(* Logix 5000 AddOnInstructionDefinition export Banner_QS18E_Param_v3; software revision 30.00; part 2 of 3 *)
(* tags used below, declared in another part *)
   QS18E : Banner_QS18E_v3;
   Port_Data : Banner_IOL_Port_v2;
   Port : DINT;
   Sensor_Type : DINT;   // 1 = D, DV, LP, CV, & FP models, 2 = EV or E models, 3 = RV or R models.
   Local_Control : DINT;
   Command_Being_Processed : BOOL;
   Update_Archive : BOOL;
   Index_Write_Inprocess : INT;
   Index_Write_Control : INT;
   Inprocess_Index : DINT;
(* Banner_QS18E_Param_v3, continued *)

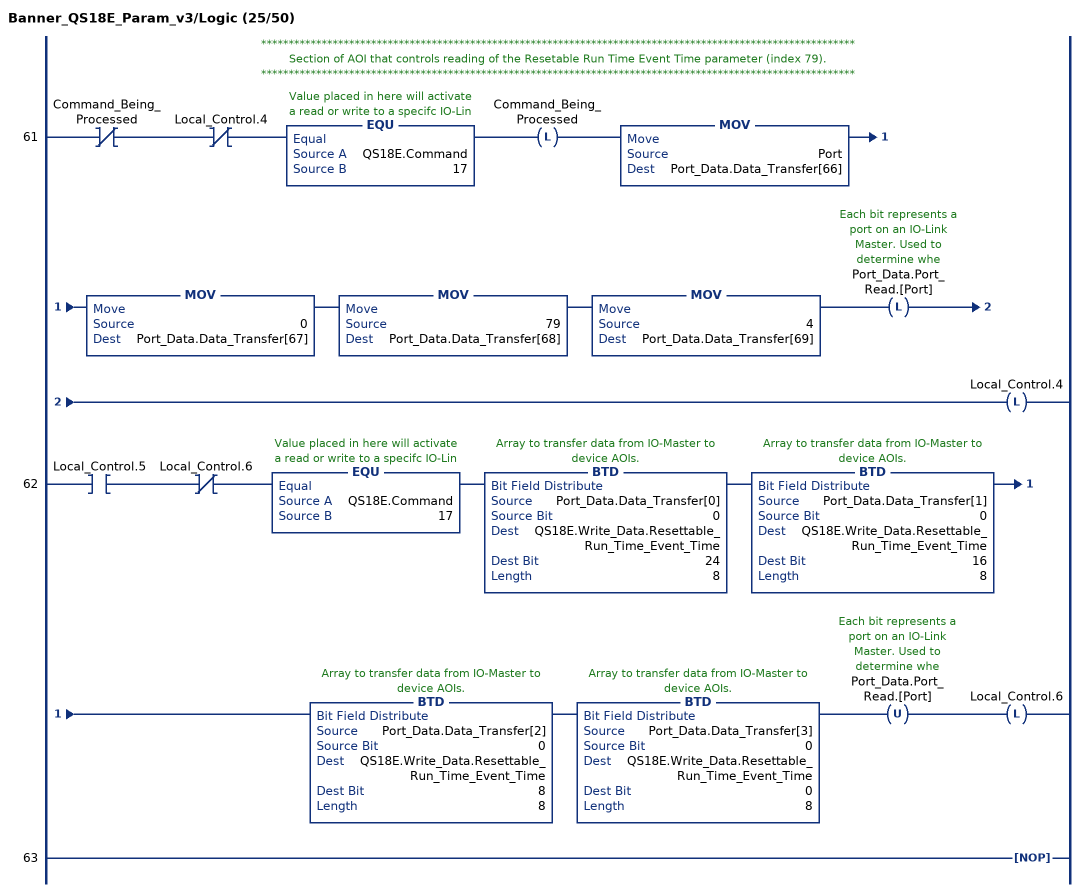
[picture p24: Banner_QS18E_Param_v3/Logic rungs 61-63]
   // ************************************************************************************************************
   // Section of AOI that controls reading of the Resetable Run Time Event Time parameter (index 79).
   // ************************************************************************************************************
   61: XIO(Command_Being_Processed)XIO(Local_Control.4)EQU(QS18E.Command,17)OTL(Command_Being_Processed)MOV(Port,Port_Data.Data_Transfer[66])MOV(0,Port_Data.Data_Transfer[67])MOV(79,Port_Data.Data_Transfer[68])MOV(4,Port_Data.Data_Transfer[69])OTL(Port_Data.Port_Read.[Port])OTL(Local_Control.4);
   62: XIC(Local_Control.5)XIO(Local_Control.6)EQU(QS18E.Command,17)BTD(Port_Data.Data_Transfer[0],0,QS18E.Write_Data.Resettable_Run_Time_Event_Time,24,8)BTD(Port_Data.Data_Transfer[1],0,QS18E.Write_Data.Resettable_Run_Time_Event_Time,16,8)BTD(Port_Data.Data_Transfer[2],0,QS18E.Write_Data.Resettable_Run_Time_Event_Time,8,8)BTD(Port_Data.Data_Transfer[3],0,QS18E.Write_Data.Resettable_Run_Time_Event_Time,0,8)OTU(Port_Data.Port_Read.[Port])OTL(Local_Control.6);
   63: NOP();
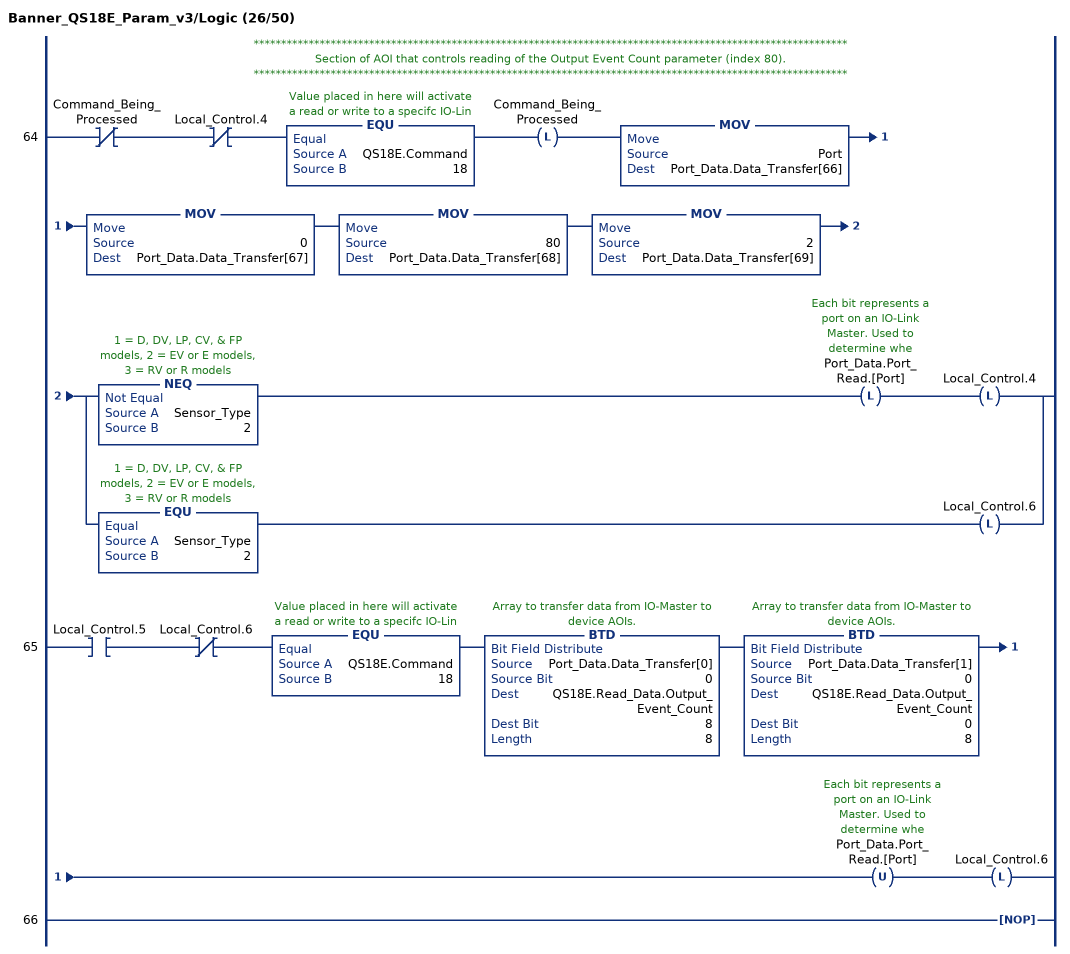
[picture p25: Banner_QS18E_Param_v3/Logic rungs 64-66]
   // ************************************************************************************************************
   // Section of AOI that controls reading of the Output Event Count parameter (index 80).
   // ************************************************************************************************************
   64: XIO(Command_Being_Processed)XIO(Local_Control.4)EQU(QS18E.Command,18)OTL(Command_Being_Processed)MOV(Port,Port_Data.Data_Transfer[66])MOV(0,Port_Data.Data_Transfer[67])MOV(80,Port_Data.Data_Transfer[68])MOV(2,Port_Data.Data_Transfer[69])[NEQ(Sensor_Type,2) OTL(Port_Data.Port_Read.[Port]) OTL(Local_Control.4) ,EQU(Sensor_Type,2) OTL(Local_Control.6) ];
   65: XIC(Local_Control.5)XIO(Local_Control.6)EQU(QS18E.Command,18)BTD(Port_Data.Data_Transfer[0],0,QS18E.Read_Data.Output_Event_Count,8,8)BTD(Port_Data.Data_Transfer[1],0,QS18E.Read_Data.Output_Event_Count,0,8)OTU(Port_Data.Port_Read.[Port])OTL(Local_Control.6);
   66: NOP();
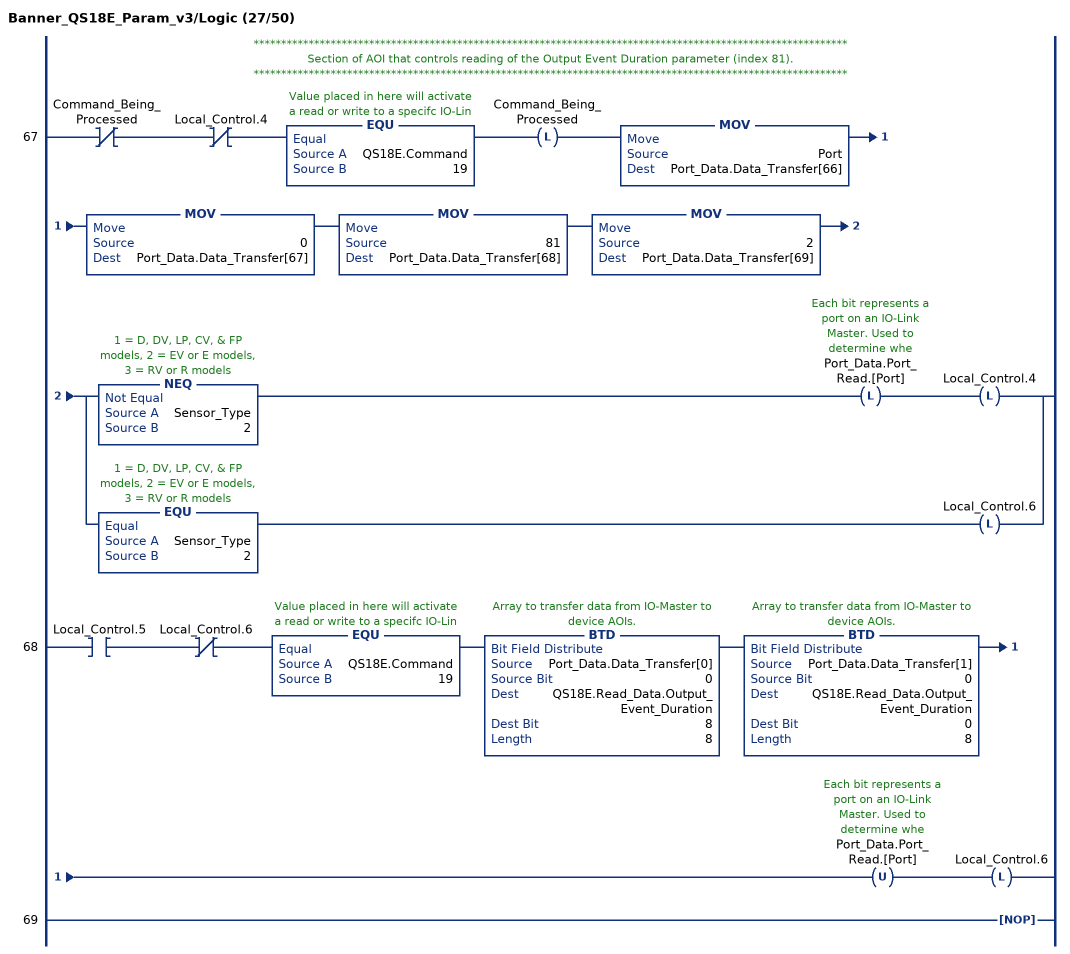
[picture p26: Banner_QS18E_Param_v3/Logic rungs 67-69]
   // ************************************************************************************************************
   // Section of AOI that controls reading of the Output Event Duration parameter (index 81).
   // ************************************************************************************************************
   67: XIO(Command_Being_Processed)XIO(Local_Control.4)EQU(QS18E.Command,19)OTL(Command_Being_Processed)MOV(Port,Port_Data.Data_Transfer[66])MOV(0,Port_Data.Data_Transfer[67])MOV(81,Port_Data.Data_Transfer[68])MOV(2,Port_Data.Data_Transfer[69])[NEQ(Sensor_Type,2) OTL(Port_Data.Port_Read.[Port]) OTL(Local_Control.4) ,EQU(Sensor_Type,2) OTL(Local_Control.6) ];
   68: XIC(Local_Control.5)XIO(Local_Control.6)EQU(QS18E.Command,19)BTD(Port_Data.Data_Transfer[0],0,QS18E.Read_Data.Output_Event_Duration,8,8)BTD(Port_Data.Data_Transfer[1],0,QS18E.Read_Data.Output_Event_Duration,0,8)OTU(Port_Data.Port_Read.[Port])OTL(Local_Control.6);
   69: NOP();
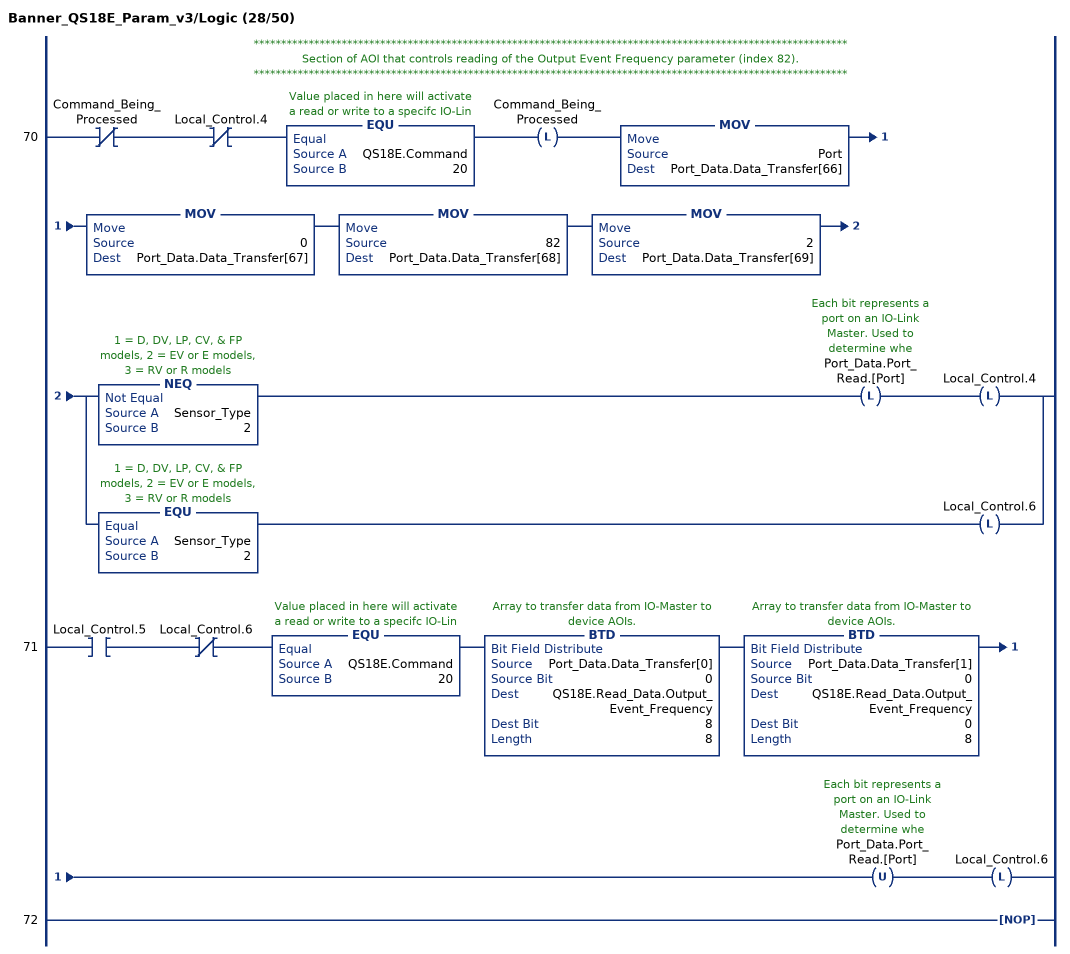
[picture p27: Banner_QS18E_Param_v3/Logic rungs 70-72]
   // ************************************************************************************************************
   // Section of AOI that controls reading of the Output Event Frequency parameter (index 82).
   // ************************************************************************************************************
   70: XIO(Command_Being_Processed)XIO(Local_Control.4)EQU(QS18E.Command,20)OTL(Command_Being_Processed)MOV(Port,Port_Data.Data_Transfer[66])MOV(0,Port_Data.Data_Transfer[67])MOV(82,Port_Data.Data_Transfer[68])MOV(2,Port_Data.Data_Transfer[69])[NEQ(Sensor_Type,2) OTL(Port_Data.Port_Read.[Port]) OTL(Local_Control.4) ,EQU(Sensor_Type,2) OTL(Local_Control.6) ];
   71: XIC(Local_Control.5)XIO(Local_Control.6)EQU(QS18E.Command,20)BTD(Port_Data.Data_Transfer[0],0,QS18E.Read_Data.Output_Event_Frequency,8,8)BTD(Port_Data.Data_Transfer[1],0,QS18E.Read_Data.Output_Event_Frequency,0,8)OTU(Port_Data.Port_Read.[Port])OTL(Local_Control.6);
   72: NOP();
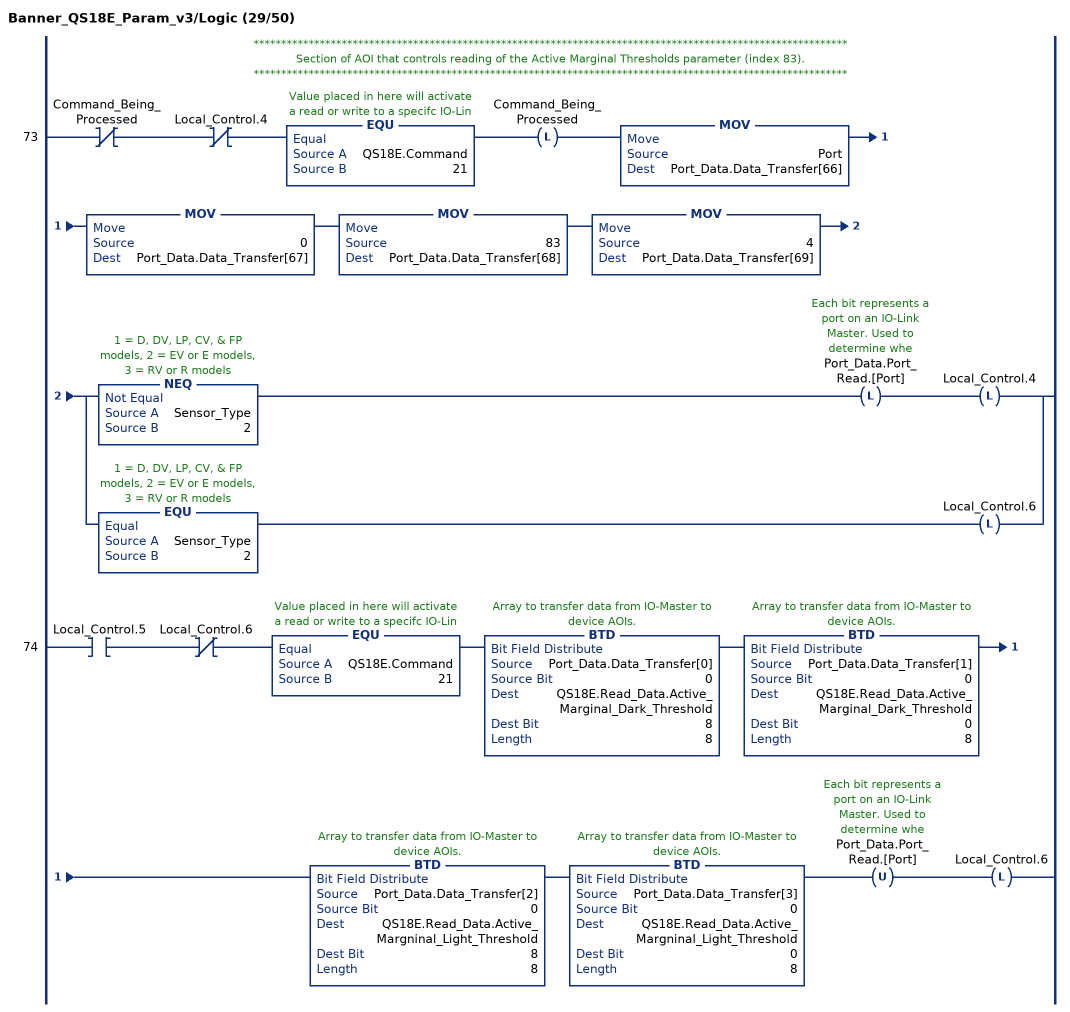
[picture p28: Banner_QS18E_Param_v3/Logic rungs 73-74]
   // ************************************************************************************************************
   // Section of AOI that controls reading of the Active Marginal Thresholds parameter (index 83).
   // ************************************************************************************************************
   73: XIO(Command_Being_Processed)XIO(Local_Control.4)EQU(QS18E.Command,21)OTL(Command_Being_Processed)MOV(Port,Port_Data.Data_Transfer[66])MOV(0,Port_Data.Data_Transfer[67])MOV(83,Port_Data.Data_Transfer[68])MOV(4,Port_Data.Data_Transfer[69])[NEQ(Sensor_Type,2) OTL(Port_Data.Port_Read.[Port]) OTL(Local_Control.4) ,EQU(Sensor_Type,2) OTL(Local_Control.6) ];
   74: XIC(Local_Control.5)XIO(Local_Control.6)EQU(QS18E.Command,21)BTD(Port_Data.Data_Transfer[0],0,QS18E.Read_Data.Active_Marginal_Dark_Threshold,8,8)BTD(Port_Data.Data_Transfer[1],0,QS18E.Read_Data.Active_Marginal_Dark_Threshold,0,8)BTD(Port_Data.Data_Transfer[2],0,QS18E.Read_Data.Active_Margninal_Light_Threshold,8,8)BTD(Port_Data.Data_Transfer[3],0,QS18E.Read_Data.Active_Margninal_Light_Threshold,0,8)OTU(Port_Data.Port_Read.[Port])OTL(Local_Control.6);
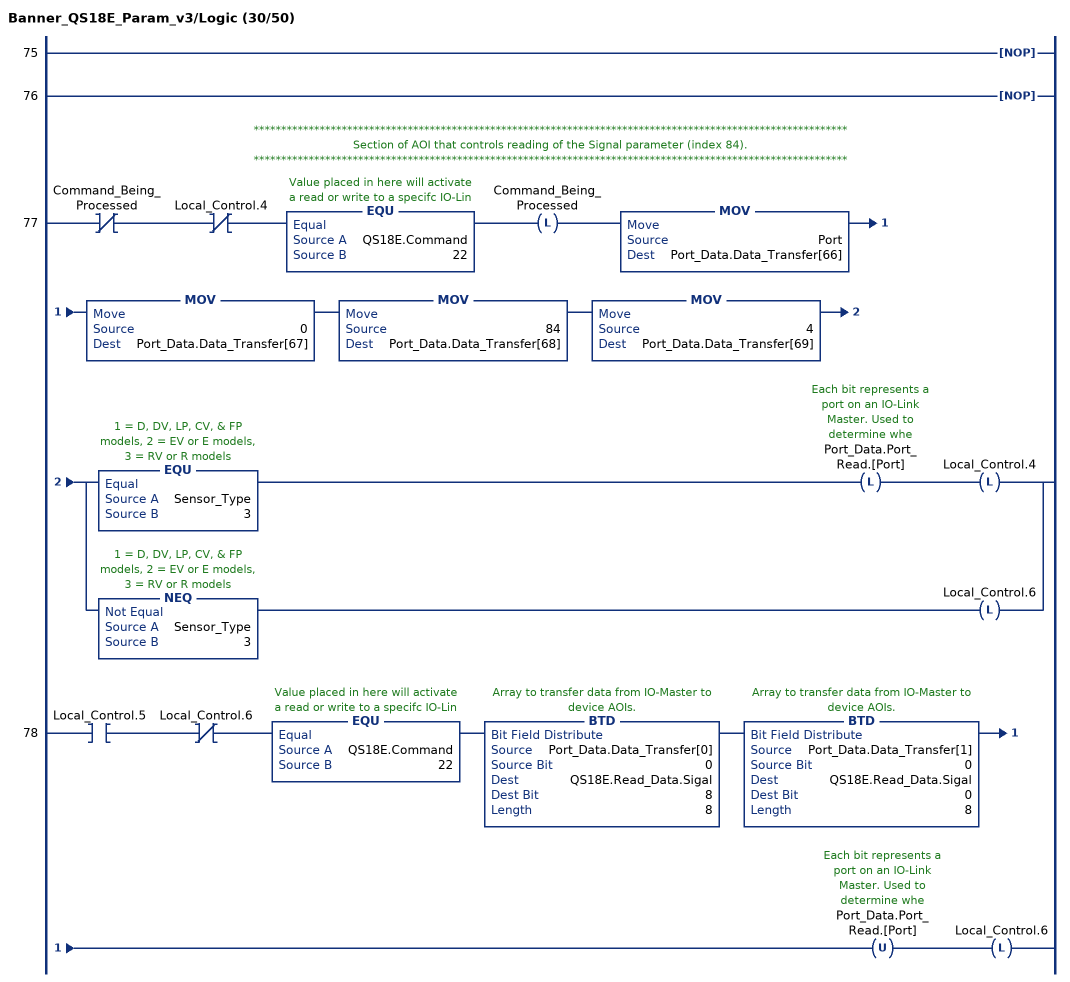
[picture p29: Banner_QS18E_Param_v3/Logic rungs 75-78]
   75: NOP();
   76: NOP();
   // ************************************************************************************************************
   // Section of AOI that controls reading of the Signal parameter (index 84).
   // ************************************************************************************************************
   77: XIO(Command_Being_Processed)XIO(Local_Control.4)EQU(QS18E.Command,22)OTL(Command_Being_Processed)MOV(Port,Port_Data.Data_Transfer[66])MOV(0,Port_Data.Data_Transfer[67])MOV(84,Port_Data.Data_Transfer[68])MOV(4,Port_Data.Data_Transfer[69])[EQU(Sensor_Type,3) OTL(Port_Data.Port_Read.[Port]) OTL(Local_Control.4) ,NEQ(Sensor_Type,3) OTL(Local_Control.6) ];
   78: XIC(Local_Control.5)XIO(Local_Control.6)EQU(QS18E.Command,22)BTD(Port_Data.Data_Transfer[0],0,QS18E.Read_Data.Sigal,8,8)BTD(Port_Data.Data_Transfer[1],0,QS18E.Read_Data.Sigal,0,8)OTU(Port_Data.Port_Read.[Port])OTL(Local_Control.6);
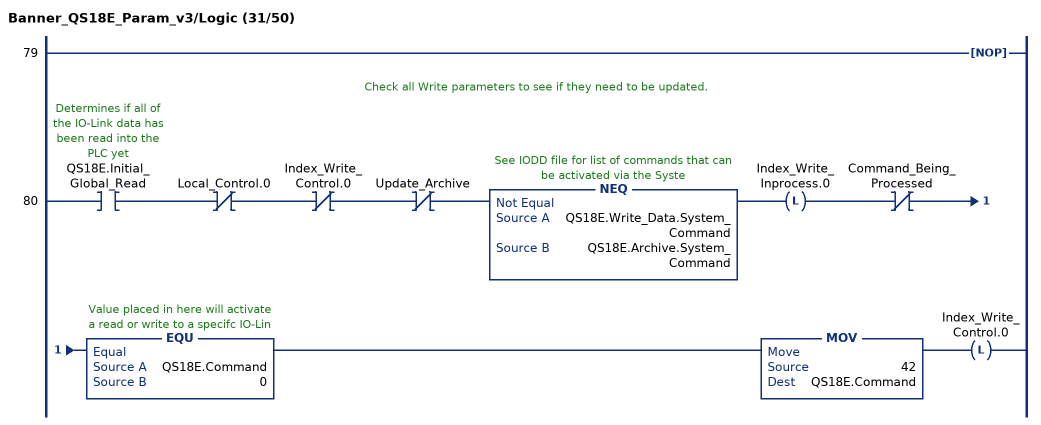
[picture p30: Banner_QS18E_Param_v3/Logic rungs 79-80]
   79: NOP();
   // Check all Write parameters to see if they need to be updated.
   80: XIC(QS18E.Initial_Global_Read)XIO(Local_Control.0)XIO(Index_Write_Control.0)XIO(Update_Archive)NEQ(QS18E.Write_Data.System_Command,QS18E.Archive.System_Command)OTL(Index_Write_Inprocess.0)XIO(Command_Being_Processed)EQU(QS18E.Command,0)MOV(42,QS18E.Command)OTL(Index_Write_Control.0);
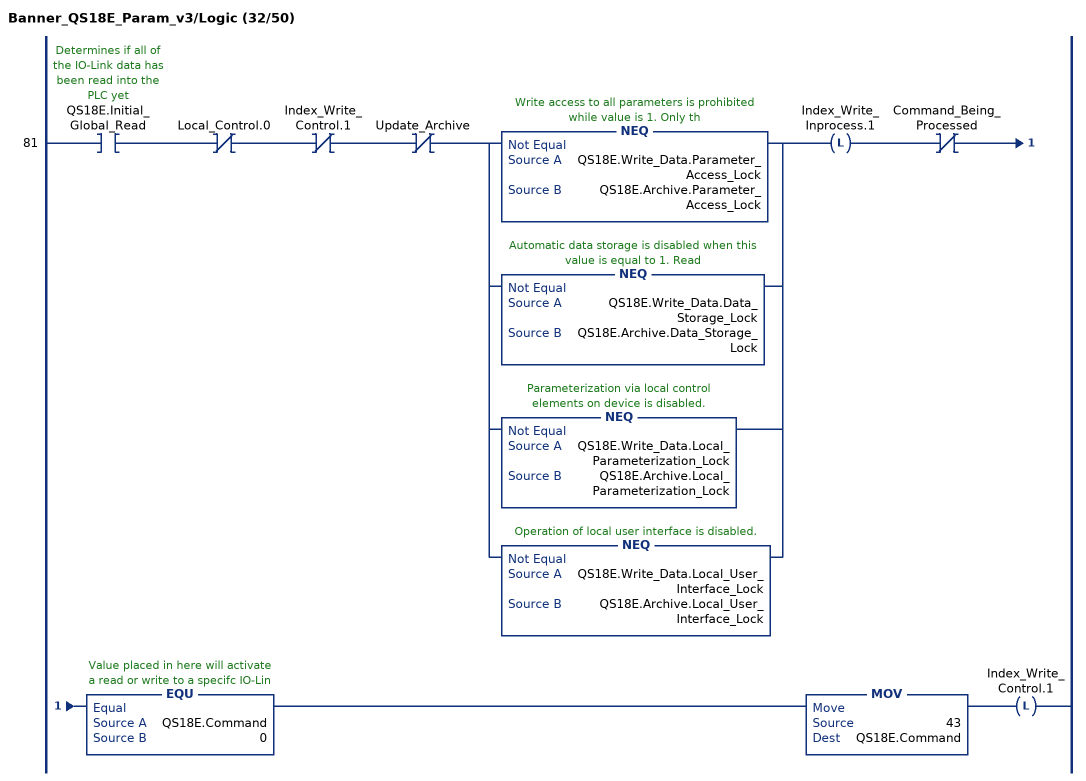
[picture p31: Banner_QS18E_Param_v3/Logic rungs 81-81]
   81: XIC(QS18E.Initial_Global_Read)XIO(Local_Control.0)XIO(Index_Write_Control.1)XIO(Update_Archive)[NEQ(QS18E.Write_Data.Parameter_Access_Lock,QS18E.Archive.Parameter_Access_Lock) ,NEQ(QS18E.Write_Data.Data_Storage_Lock,QS18E.Archive.Data_Storage_Lock) ,NEQ(QS18E.Write_Data.Local_Parameterization_Lock,QS18E.Archive.Local_Parameterization_Lock) ,NEQ(QS18E.Write_Data.Local_User_Interface_Lock,QS18E.Archive.Local_User_Interface_Lock) ]OTL(Index_Write_Inprocess.1)XIO(Command_Being_Processed)EQU(QS18E.Command,0)MOV(43,QS18E.Command)OTL(Index_Write_Control.1);
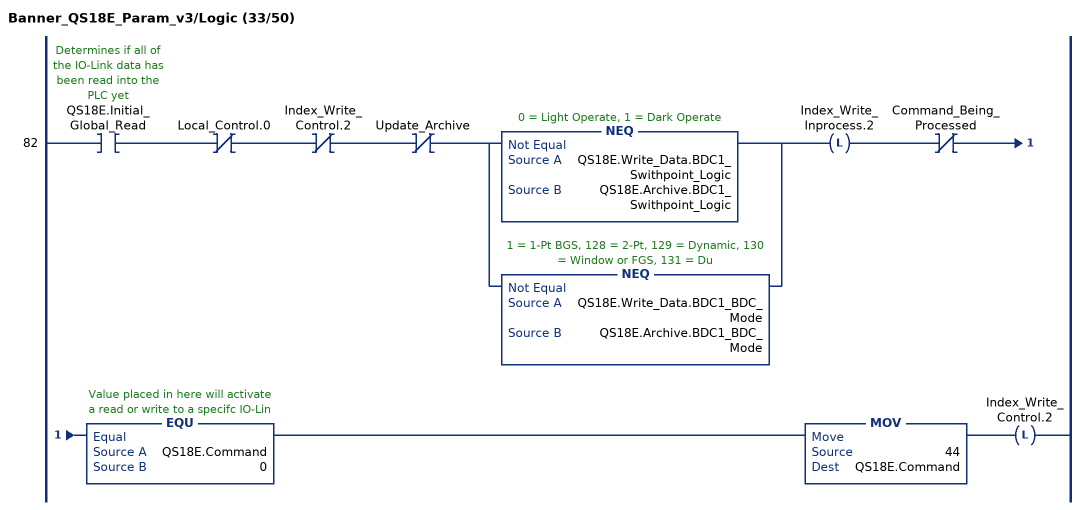
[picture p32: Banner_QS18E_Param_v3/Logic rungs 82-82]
   82: XIC(QS18E.Initial_Global_Read)XIO(Local_Control.0)XIO(Index_Write_Control.2)XIO(Update_Archive)[NEQ(QS18E.Write_Data.BDC1_Swithpoint_Logic,QS18E.Archive.BDC1_Swithpoint_Logic) ,NEQ(QS18E.Write_Data.BDC1_BDC_Mode,QS18E.Archive.BDC1_BDC_Mode) ]OTL(Index_Write_Inprocess.2)XIO(Command_Being_Processed)EQU(QS18E.Command,0)MOV(44,QS18E.Command)OTL(Index_Write_Control.2);
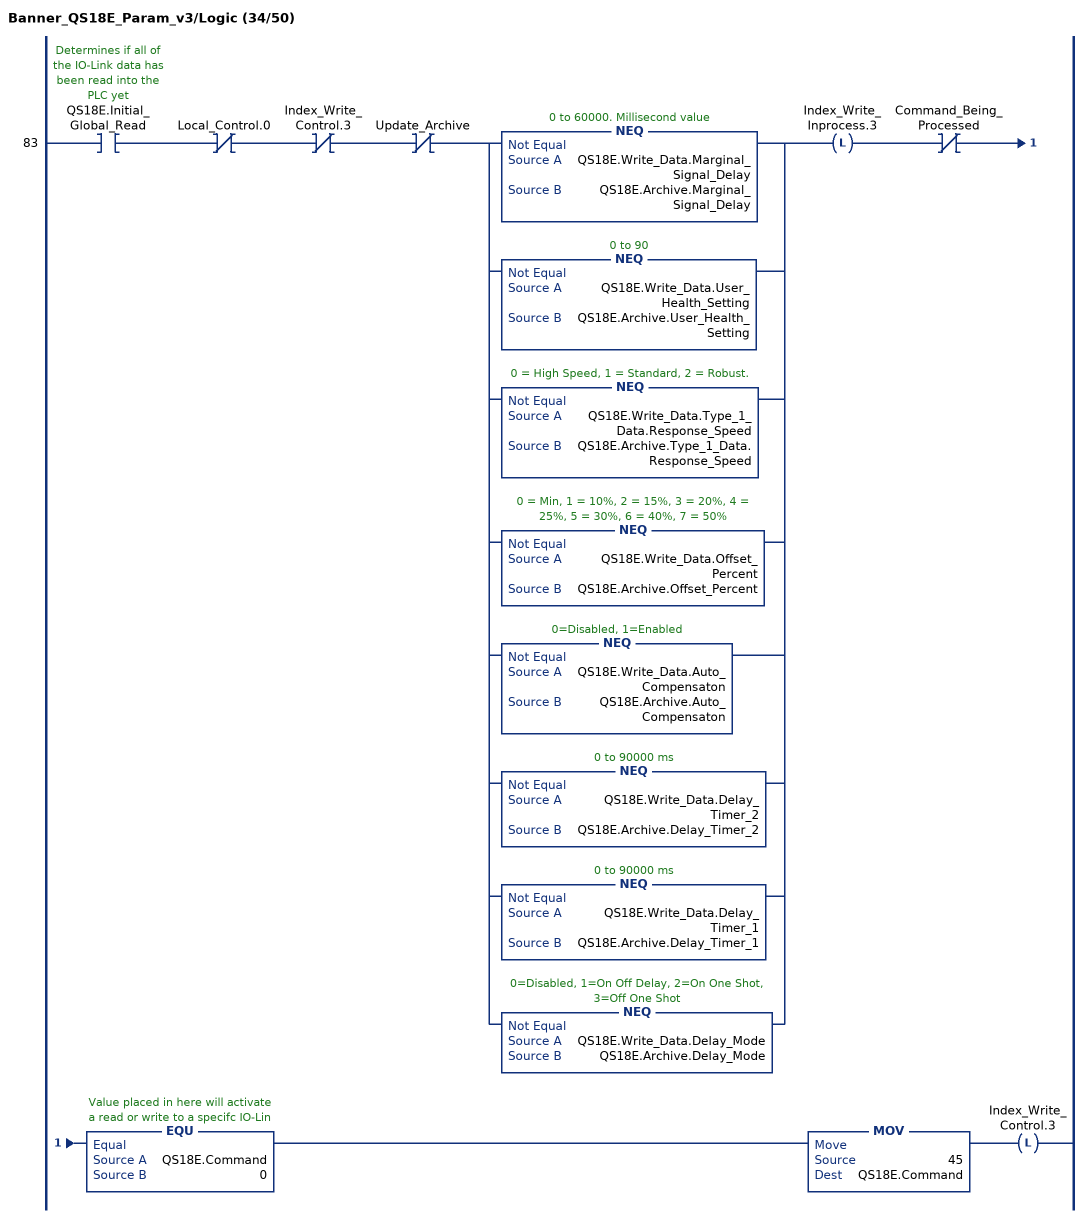
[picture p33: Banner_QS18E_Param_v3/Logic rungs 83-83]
   83: XIC(QS18E.Initial_Global_Read)XIO(Local_Control.0)XIO(Index_Write_Control.3)XIO(Update_Archive)[NEQ(QS18E.Write_Data.Marginal_Signal_Delay,QS18E.Archive.Marginal_Signal_Delay) ,NEQ(QS18E.Write_Data.User_Health_Setting,QS18E.Archive.User_Health_Setting) ,NEQ(QS18E.Write_Data.Type_1_Data.Response_Speed,QS18E.Archive.Type_1_Data.Response_Speed) ,NEQ(QS18E.Write_Data.Offset_Percent,QS18E.Archive.Offset_Percent) ,NEQ(QS18E.Write_Data.Auto_Compensaton,QS18E.Archive.Auto_Compensaton) ,NEQ(QS18E.Write_Data.Delay_Timer_2,QS18E.Archive.Delay_Timer_2) ,NEQ(QS18E.Write_Data.Delay_Timer_1,QS18E.Archive.Delay_Timer_1) ,NEQ(QS18E.Write_Data.Delay_Mode,QS18E.Archive.Delay_Mode) ]OTL(Index_Write_Inprocess.3)XIO(Command_Being_Processed)EQU(QS18E.Command,0)MOV(45,QS18E.Command)OTL(Index_Write_Control.3);
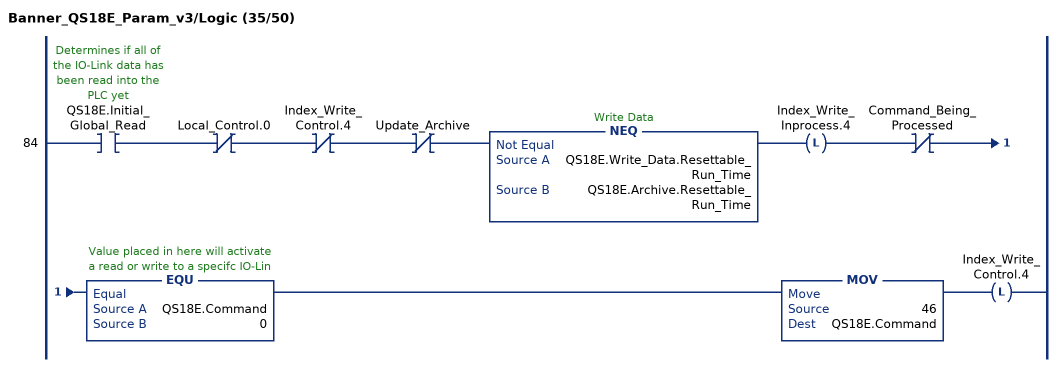
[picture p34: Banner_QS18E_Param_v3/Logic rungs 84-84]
   84: XIC(QS18E.Initial_Global_Read)XIO(Local_Control.0)XIO(Index_Write_Control.4)XIO(Update_Archive)NEQ(QS18E.Write_Data.Resettable_Run_Time,QS18E.Archive.Resettable_Run_Time)OTL(Index_Write_Inprocess.4)XIO(Command_Being_Processed)EQU(QS18E.Command,0)MOV(46,QS18E.Command)OTL(Index_Write_Control.4);
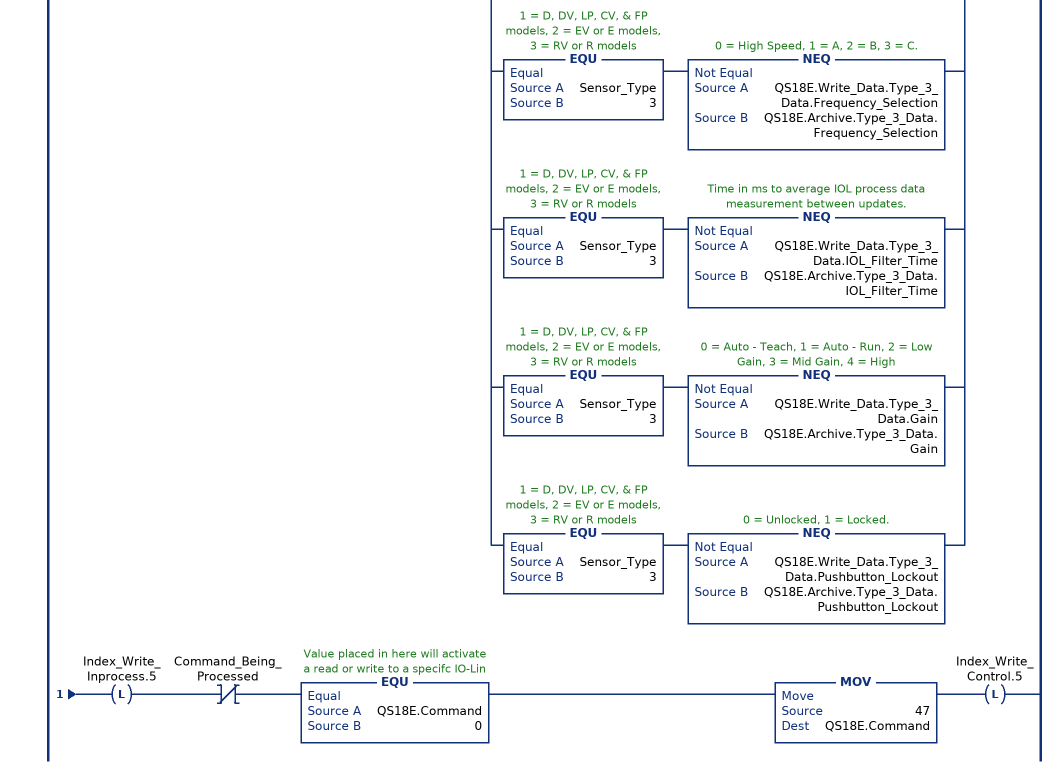
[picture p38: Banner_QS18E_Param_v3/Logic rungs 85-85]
   85: XIC(QS18E.Initial_Global_Read)XIO(Local_Control.0)XIO(Index_Write_Control.5)XIO(Update_Archive)[EQU(Sensor_Type,1) NEQ(QS18E.Write_Data.Type_1_Data.Polarity_of_Pins_2_and_4,QS18E.Archive.Type_1_Data.Polarity_of_Pins_2_and_4) ,EQU(Sensor_Type,1) NEQ(QS18E.Write_Data.Type_1_Data.Pin_2_Config,QS18E.Archive.Type_1_Data.Pin_2_Config) ,EQU(Sensor_Type,1) NEQ(QS18E.Write_Data.Type_1_Data.Process_Data_Input_Config,QS18E.Archive.Type_1_Data.Process_Data_Input_Config) ,EQU(Sensor_Type,1) NEQ(QS18E.Write_Data.Type_1_Data.Marginal_Mode,QS18E.Archive.Type_1_Data.Marginal_Mode) ,EQU(Sensor_Type,1) NEQ(QS18E.Write_Data.Type_1_Data.User_Marginal_Light,QS18E.Archive.Type_1_Data.User_Marginal_Light) ,EQU(Sensor_Type,1) NEQ(QS18E.Write_Data.Type_1_Data.User_Marginal_Dark,QS18E.Archive.Type_1_Data.User_Marginal_Dark) ,EQU(Sensor_Type,1) NEQ(QS18E.Write_Data.Type_1_Data.LED_Power,QS18E.Archive.Type_1_Data.LED_Power) ,EQU(Sensor_Type,2) NEQ(QS18E.Write_Data.Type_2_Data.Polarity_of_Pins_2_and_4,QS18E.Archive.Type_2_Data.Polarity_of_Pins_2_and_4) ,EQU(Sensor_Type,2) NEQ(QS18E.Write_Data.Type_2_Data.Pin_2_Config,QS18E.Archive.Type_2_Data.Pin_2_Config) ,EQU(Sensor_Type,2) NEQ(QS18E.Write_Data.Type_2_Data.Frequency_Selection,QS18E.Archive.Type_2_Data.Frequency_Selection) ,EQU(Sensor_Type,2) NEQ(QS18E.Write_Data.Type_2_Data.Power_Level,QS18E.Archive.Type_2_Data.Power_Level) ,EQU(Sensor_Type,2) NEQ(QS18E.Write_Data.Type_2_Data.Pushbutton_Lockout,QS18E.Archive.Type_2_Data.Pushbutton_Lockout) ,EQU(Sensor_Type,3) NEQ(QS18E.Write_Data.Type_3_Data.Polarity_of_Pins_2_and_4,QS18E.Archive.Type_3_Data.Polarity_of_Pins_2_and_4) ,EQU(Sensor_Type,3) NEQ(QS18E.Write_Data.Type_3_Data.Pin_2_Config,QS18E.Archive.Type_3_Data.Pin_2_Config) ,EQU(Sensor_Type,3) NEQ(QS18E.Write_Data.Type_3_Data.Process_Data_Input_Config,QS18E.Archive.Type_3_Data.Process_Data_Input_Config) ,EQU(Sensor_Type,3) NEQ(QS18E.Write_Data.Type_3_Data.Marginal_Mode,QS18E.Archive.Type_3_Data.Marginal_Mode) ,EQU(Sensor_Type,3) NEQ(QS18E.Write_Data.Type_3_Data.User_Marginal_Light,QS18E.Archive.Type_3_Data.User_Marginal_Light) ,EQU(Sensor_Type,3) NEQ(QS18E.Write_Data.Type_3_Data.User_Marginal_Dark,QS18E.Archive.Type_3_Data.User_Marginal_Dark) ,EQU(Sensor_Type,3) NEQ(QS18E.Write_Data.Type_3_Data.Frequency_Selection,QS18E.Archive.Type_3_Data.Frequency_Selection) ,EQU(Sensor_Type,3) NEQ(QS18E.Write_Data.Type_3_Data.IOL_Filter_Time,QS18E.Archive.Type_3_Data.IOL_Filter_Time) ,EQU(Sensor_Type,3) NEQ(QS18E.Write_Data.Type_3_Data.Gain,QS18E.Archive.Type_3_Data.Gain) ,EQU(Sensor_Type,3) NEQ(QS18E.Write_Data.Type_3_Data.Pushbutton_Lockout,QS18E.Archive.Type_3_Data.Pushbutton_Lockout) ]OTL(Index_Write_Inprocess.5)XIO(Command_Being_Processed)EQU(QS18E.Command,0)MOV(47,QS18E.Command)OTL(Index_Write_Control.5);
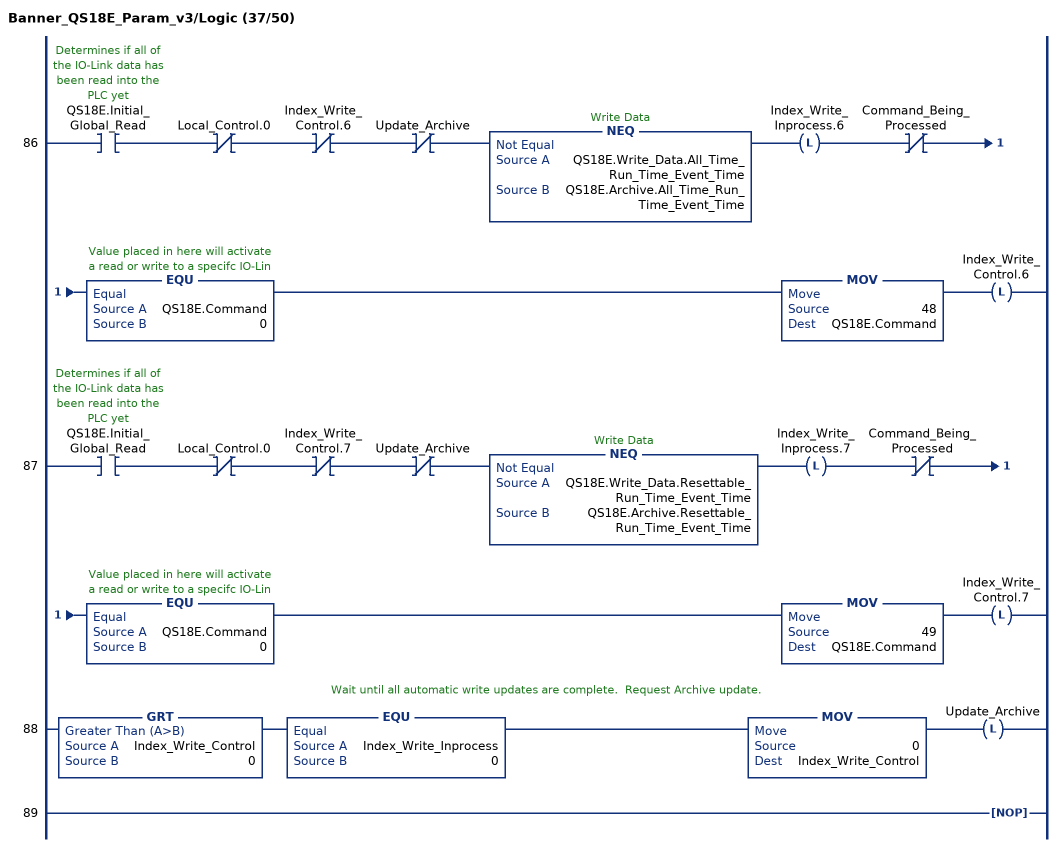
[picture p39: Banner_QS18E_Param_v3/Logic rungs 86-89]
   86: XIC(QS18E.Initial_Global_Read)XIO(Local_Control.0)XIO(Index_Write_Control.6)XIO(Update_Archive)NEQ(QS18E.Write_Data.All_Time_Run_Time_Event_Time,QS18E.Archive.All_Time_Run_Time_Event_Time)OTL(Index_Write_Inprocess.6)XIO(Command_Being_Processed)EQU(QS18E.Command,0)MOV(48,QS18E.Command)OTL(Index_Write_Control.6);
   87: XIC(QS18E.Initial_Global_Read)XIO(Local_Control.0)XIO(Index_Write_Control.7)XIO(Update_Archive)NEQ(QS18E.Write_Data.Resettable_Run_Time_Event_Time,QS18E.Archive.Resettable_Run_Time_Event_Time)OTL(Index_Write_Inprocess.7)XIO(Command_Being_Processed)EQU(QS18E.Command,0)MOV(49,QS18E.Command)OTL(Index_Write_Control.7);
   // Wait until all automatic write updates are complete.  Request Archive update.
   88: GRT(Index_Write_Control,0)EQU(Index_Write_Inprocess,0)MOV(0,Index_Write_Control)OTL(Update_Archive);
   89: NOP();
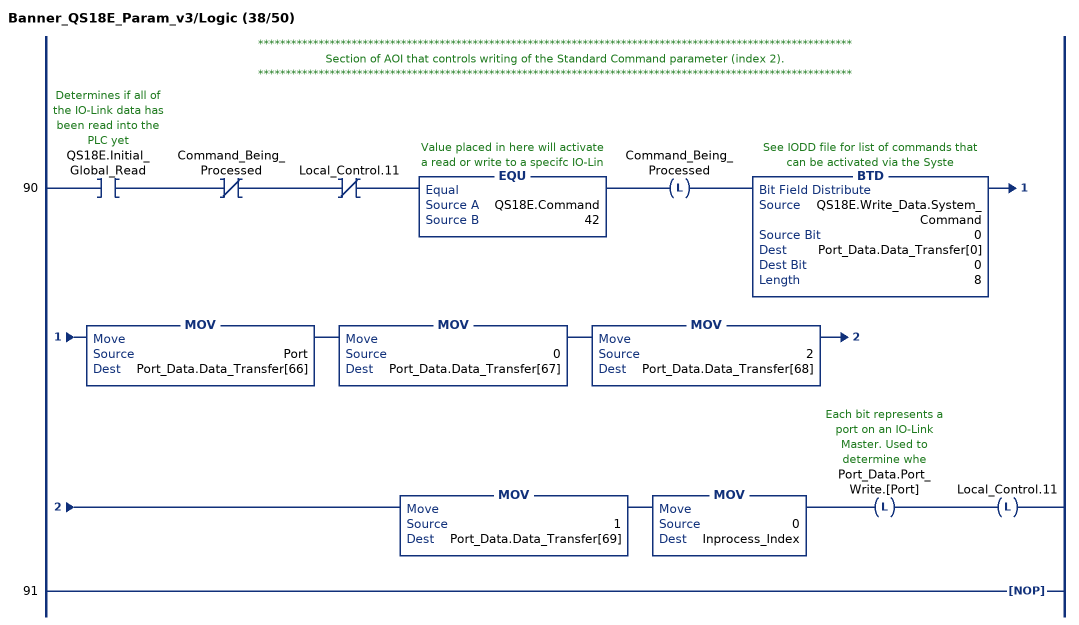
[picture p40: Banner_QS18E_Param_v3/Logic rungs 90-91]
   // ************************************************************************************************************
   // Section of AOI that controls writing of the Standard Command parameter (index 2).
   // ************************************************************************************************************
   90: XIC(QS18E.Initial_Global_Read)XIO(Command_Being_Processed)XIO(Local_Control.11)EQU(QS18E.Command,42)OTL(Command_Being_Processed)BTD(QS18E.Write_Data.System_Command,0,Port_Data.Data_Transfer[0],0,8)MOV(Port,Port_Data.Data_Transfer[66])MOV(0,Port_Data.Data_Transfer[67])MOV(2,Port_Data.Data_Transfer[68])MOV(1,Port_Data.Data_Transfer[69])MOV(0,Inprocess_Index)OTL(Port_Data.Port_Write.[Port])OTL(Local_Control.11);
   91: NOP();
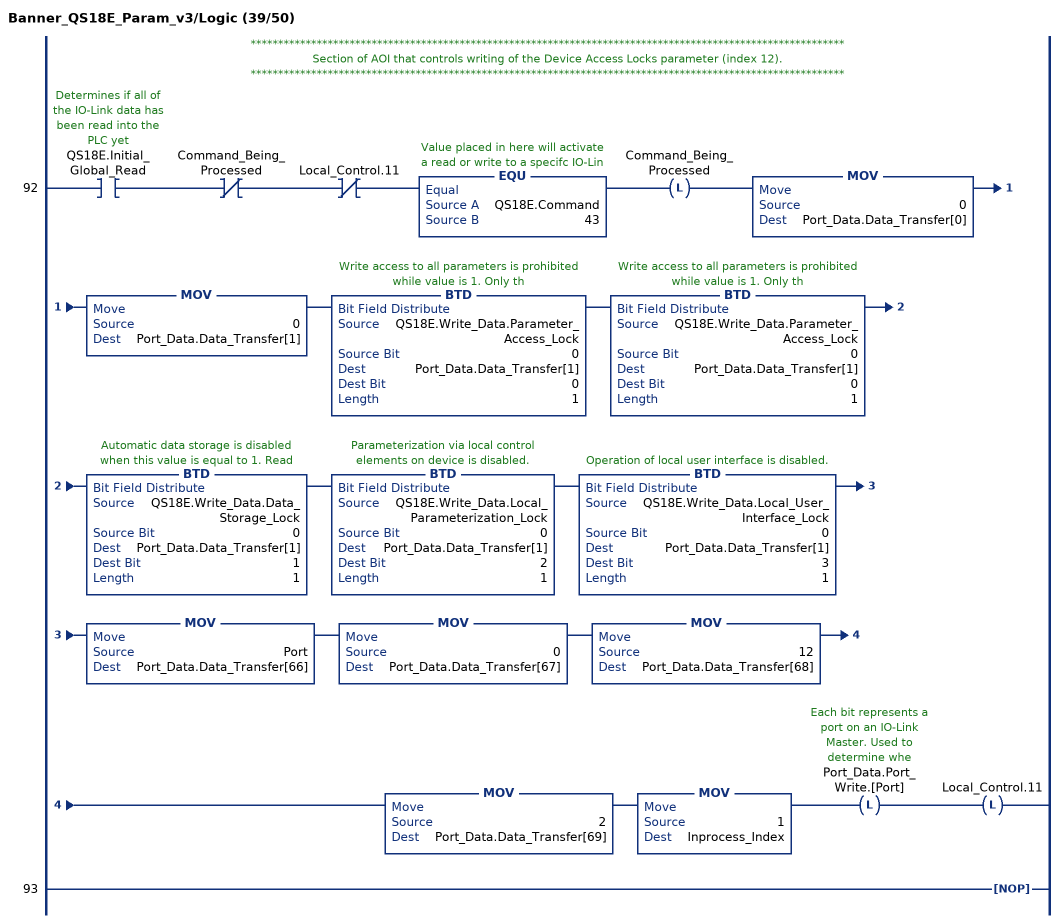
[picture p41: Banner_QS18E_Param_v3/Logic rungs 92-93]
   // ************************************************************************************************************
   // Section of AOI that controls writing of the Device Access Locks parameter (index 12).
   // ************************************************************************************************************
   92: XIC(QS18E.Initial_Global_Read)XIO(Command_Being_Processed)XIO(Local_Control.11)EQU(QS18E.Command,43)OTL(Command_Being_Processed)MOV(0,Port_Data.Data_Transfer[0])MOV(0,Port_Data.Data_Transfer[1])BTD(QS18E.Write_Data.Parameter_Access_Lock,0,Port_Data.Data_Transfer[1],0,1)BTD(QS18E.Write_Data.Parameter_Access_Lock,0,Port_Data.Data_Transfer[1],0,1)BTD(QS18E.Write_Data.Data_Storage_Lock,0,Port_Data.Data_Transfer[1],1,1)BTD(QS18E.Write_Data.Local_Parameterization_Lock,0,Port_Data.Data_Transfer[1],2,1)BTD(QS18E.Write_Data.Local_User_Interface_Lock,0,Port_Data.Data_Transfer[1],3,1)MOV(Port,Port_Data.Data_Transfer[66])MOV(0,Port_Data.Data_Transfer[67])MOV(12,Port_Data.Data_Transfer[68])MOV(2,Port_Data.Data_Transfer[69])MOV(1,Inprocess_Index)OTL(Port_Data.Port_Write.[Port])OTL(Local_Control.11);
   93: NOP();
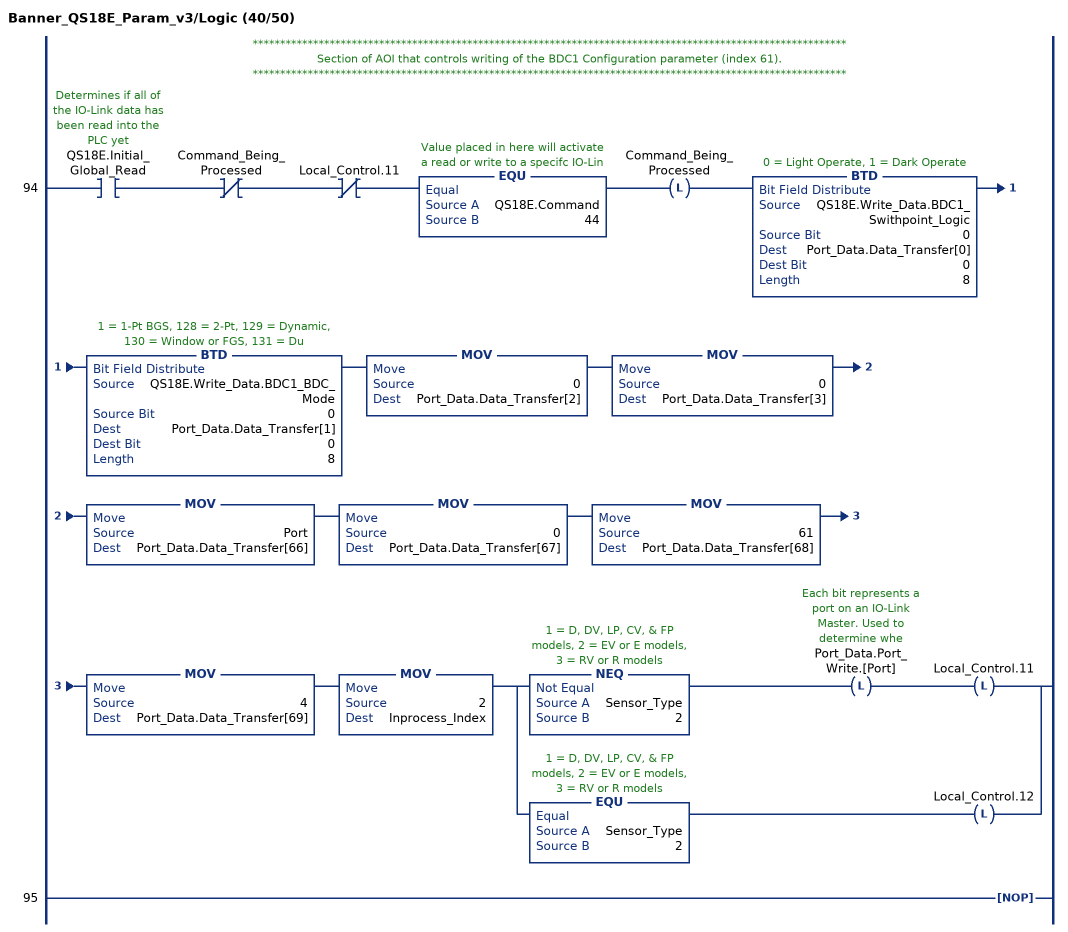
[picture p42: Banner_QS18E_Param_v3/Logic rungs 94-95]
   // ************************************************************************************************************
   // Section of AOI that controls writing of the BDC1 Configuration parameter (index 61).
   // ************************************************************************************************************
   94: XIC(QS18E.Initial_Global_Read)XIO(Command_Being_Processed)XIO(Local_Control.11)EQU(QS18E.Command,44)OTL(Command_Being_Processed)BTD(QS18E.Write_Data.BDC1_Swithpoint_Logic,0,Port_Data.Data_Transfer[0],0,8)BTD(QS18E.Write_Data.BDC1_BDC_Mode,0,Port_Data.Data_Transfer[1],0,8)MOV(0,Port_Data.Data_Transfer[2])MOV(0,Port_Data.Data_Transfer[3])MOV(Port,Port_Data.Data_Transfer[66])MOV(0,Port_Data.Data_Transfer[67])MOV(61,Port_Data.Data_Transfer[68])MOV(4,Port_Data.Data_Transfer[69])MOV(2,Inprocess_Index)[NEQ(Sensor_Type,2) OTL(Port_Data.Port_Write.[Port]) OTL(Local_Control.11) ,EQU(Sensor_Type,2) OTL(Local_Control.12) ];
   95: NOP();
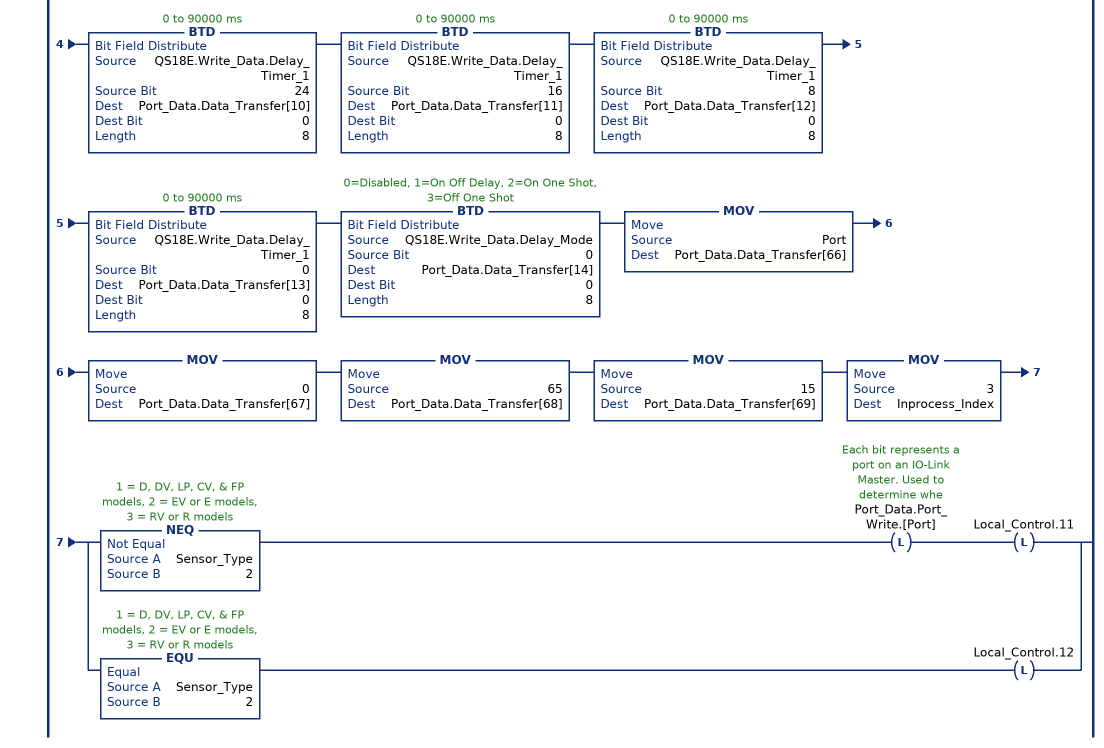
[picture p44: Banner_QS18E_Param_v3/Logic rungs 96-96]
   // ************************************************************************************************************
   // Section of AOI that controls writing of the BDC1 Vendor Specific Configuration parameter (index 65).
   // ************************************************************************************************************
   96: XIC(QS18E.Initial_Global_Read)XIO(Command_Being_Processed)XIO(Local_Control.11)EQU(QS18E.Command,45)OTL(Command_Being_Processed)BTD(QS18E.Write_Data.Marginal_Signal_Delay,8,Port_Data.Data_Transfer[0],0,8)BTD(QS18E.Write_Data.Marginal_Signal_Delay,0,Port_Data.Data_Transfer[1],0,8)BTD(QS18E.Write_Data.User_Health_Setting,0,Port_Data.Data_Transfer[2],0,8)[EQU(Sensor_Type,1) BTD(QS18E.Write_Data.Type_1_Data.Response_Speed,0,Port_Data.Data_Transfer[3],0,8) ,NEQ(Sensor_Type,1) MOV(0,Port_Data.Data_Transfer[3]) ]BTD(QS18E.Write_Data.Offset_Percent,0,Port_Data.Data_Transfer[4],0,8)BTD(QS18E.Write_Data.Auto_Compensaton,0,Port_Data.Data_Transfer[5],0,8)BTD(QS18E.Write_Data.Delay_Timer_2,24,Port_Data.Data_Transfer[6],0,8)BTD(QS18E.Write_Data.Delay_Timer_2,16,Port_Data.Data_Transfer[7],0,8)BTD(QS18E.Write_Data.Delay_Timer_2,8,Port_Data.Data_Transfer[8],0,8)BTD(QS18E.Write_Data.Delay_Timer_2,0,Port_Data.Data_Transfer[9],0,8)BTD(QS18E.Write_Data.Delay_Timer_1,24,Port_Data.Data_Transfer[10],0,8)BTD(QS18E.Write_Data.Delay_Timer_1,16,Port_Data.Data_Transfer[11],0,8)BTD(QS18E.Write_Data.Delay_Timer_1,8,Port_Data.Data_Transfer[12],0,8)BTD(QS18E.Write_Data.Delay_Timer_1,0,Port_Data.Data_Transfer[13],0,8)BTD(QS18E.Write_Data.Delay_Mode,0,Port_Data.Data_Transfer[14],0,8)MOV(Port,Port_Data.Data_Transfer[66])MOV(0,Port_Data.Data_Transfer[67])MOV(65,Port_Data.Data_Transfer[68])MOV(15,Port_Data.Data_Transfer[69])MOV(3,Inprocess_Index)[NEQ(Sensor_Type,2) OTL(Port_Data.Port_Write.[Port]) OTL(Local_Control.11) ,EQU(Sensor_Type,2) OTL(Local_Control.12) ];
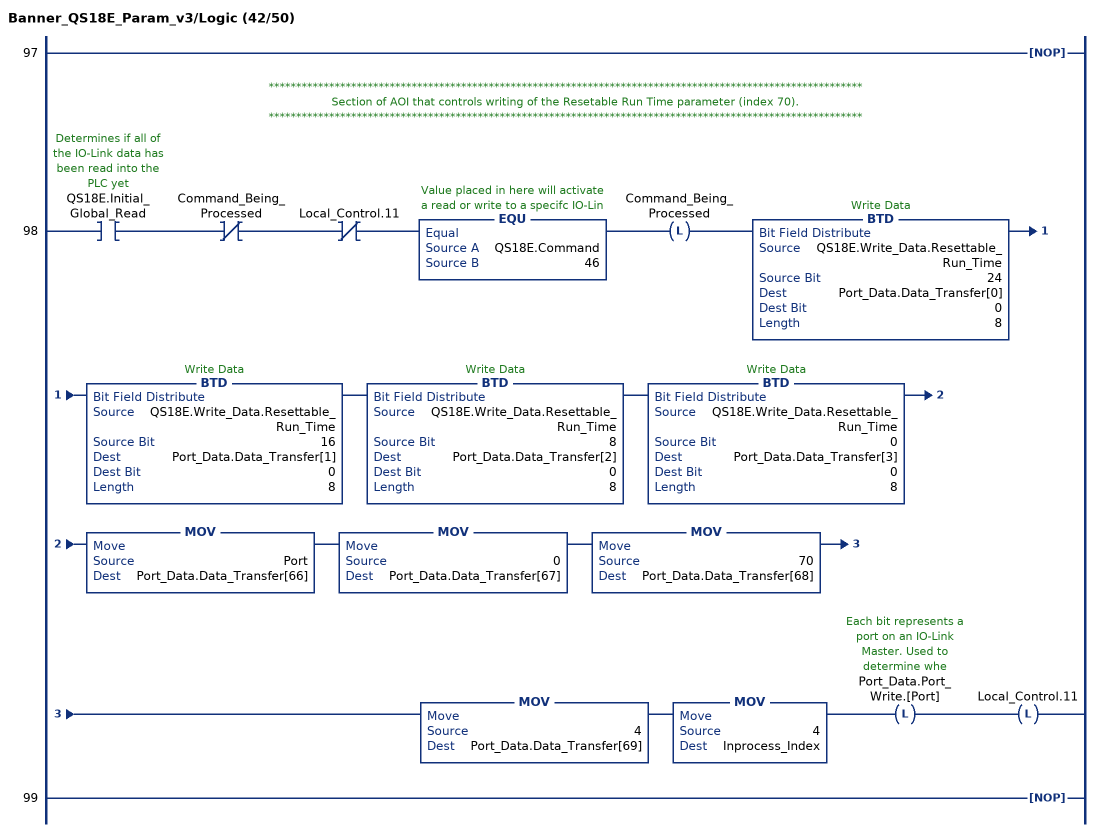
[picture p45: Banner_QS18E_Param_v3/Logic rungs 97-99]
   97: NOP();
   // ************************************************************************************************************
   // Section of AOI that controls writing of the Resetable Run Time parameter (index 70).
   // ************************************************************************************************************
   98: XIC(QS18E.Initial_Global_Read)XIO(Command_Being_Processed)XIO(Local_Control.11)EQU(QS18E.Command,46)OTL(Command_Being_Processed)BTD(QS18E.Write_Data.Resettable_Run_Time,24,Port_Data.Data_Transfer[0],0,8)BTD(QS18E.Write_Data.Resettable_Run_Time,16,Port_Data.Data_Transfer[1],0,8)BTD(QS18E.Write_Data.Resettable_Run_Time,8,Port_Data.Data_Transfer[2],0,8)BTD(QS18E.Write_Data.Resettable_Run_Time,0,Port_Data.Data_Transfer[3],0,8)MOV(Port,Port_Data.Data_Transfer[66])MOV(0,Port_Data.Data_Transfer[67])MOV(70,Port_Data.Data_Transfer[68])MOV(4,Port_Data.Data_Transfer[69])MOV(4,Inprocess_Index)OTL(Port_Data.Port_Write.[Port])OTL(Local_Control.11);
   99: NOP();
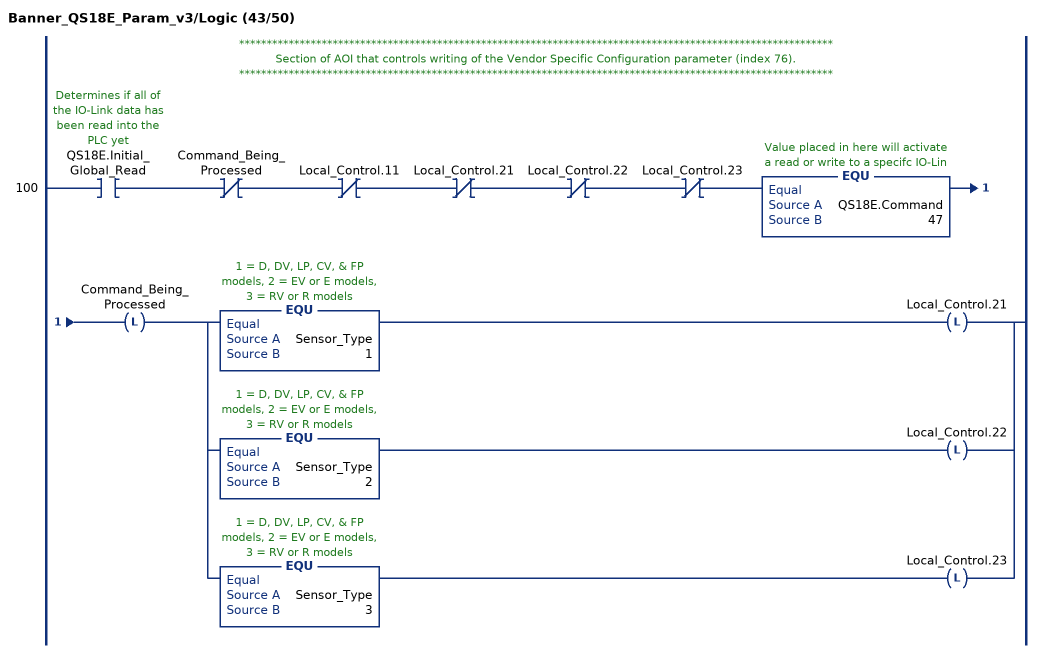
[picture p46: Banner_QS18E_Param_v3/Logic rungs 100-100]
   // ************************************************************************************************************
   // Section of AOI that controls writing of the Vendor Specific Configuration parameter (index 76).
   // ************************************************************************************************************
   100: XIC(QS18E.Initial_Global_Read)XIO(Command_Being_Processed)XIO(Local_Control.11)XIO(Local_Control.21)XIO(Local_Control.22)XIO(Local_Control.23)EQU(QS18E.Command,47)OTL(Command_Being_Processed)[EQU(Sensor_Type,1) OTL(Local_Control.21) ,EQU(Sensor_Type,2) OTL(Local_Control.22) ,EQU(Sensor_Type,3) OTL(Local_Control.23) ];
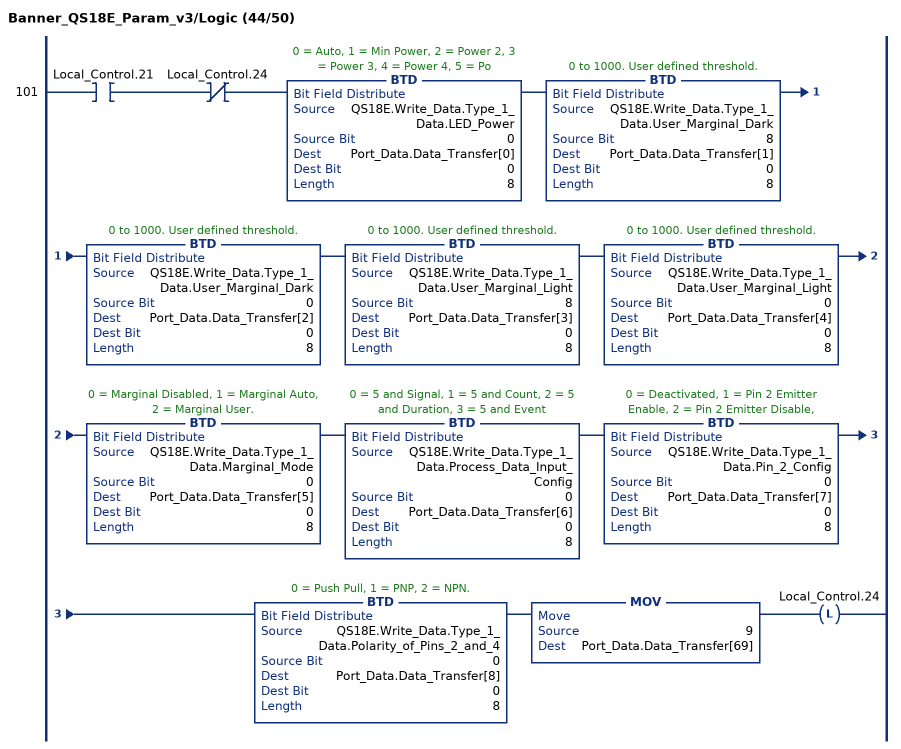
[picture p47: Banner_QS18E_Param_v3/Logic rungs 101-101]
   101: XIC(Local_Control.21)XIO(Local_Control.24)BTD(QS18E.Write_Data.Type_1_Data.LED_Power,0,Port_Data.Data_Transfer[0],0,8)BTD(QS18E.Write_Data.Type_1_Data.User_Marginal_Dark,8,Port_Data.Data_Transfer[1],0,8)BTD(QS18E.Write_Data.Type_1_Data.User_Marginal_Dark,0,Port_Data.Data_Transfer[2],0,8)BTD(QS18E.Write_Data.Type_1_Data.User_Marginal_Light,8,Port_Data.Data_Transfer[3],0,8)BTD(QS18E.Write_Data.Type_1_Data.User_Marginal_Light,0,Port_Data.Data_Transfer[4],0,8)BTD(QS18E.Write_Data.Type_1_Data.Marginal_Mode,0,Port_Data.Data_Transfer[5],0,8)BTD(QS18E.Write_Data.Type_1_Data.Process_Data_Input_Config,0,Port_Data.Data_Transfer[6],0,8)BTD(QS18E.Write_Data.Type_1_Data.Pin_2_Config,0,Port_Data.Data_Transfer[7],0,8)BTD(QS18E.Write_Data.Type_1_Data.Polarity_of_Pins_2_and_4,0,Port_Data.Data_Transfer[8],0,8)MOV(9,Port_Data.Data_Transfer[69])OTL(Local_Control.24);
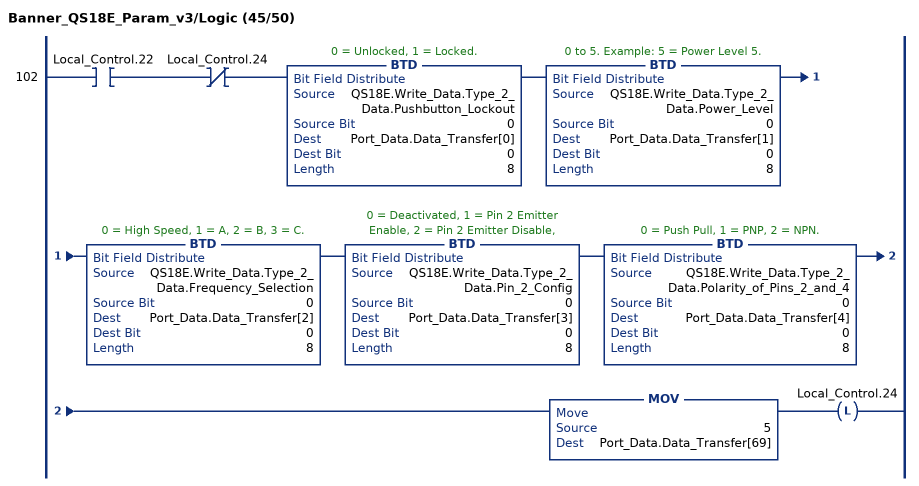
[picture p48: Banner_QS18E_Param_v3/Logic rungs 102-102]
   102: XIC(Local_Control.22)XIO(Local_Control.24)BTD(QS18E.Write_Data.Type_2_Data.Pushbutton_Lockout,0,Port_Data.Data_Transfer[0],0,8)BTD(QS18E.Write_Data.Type_2_Data.Power_Level,0,Port_Data.Data_Transfer[1],0,8)BTD(QS18E.Write_Data.Type_2_Data.Frequency_Selection,0,Port_Data.Data_Transfer[2],0,8)BTD(QS18E.Write_Data.Type_2_Data.Pin_2_Config,0,Port_Data.Data_Transfer[3],0,8)BTD(QS18E.Write_Data.Type_2_Data.Polarity_of_Pins_2_and_4,0,Port_Data.Data_Transfer[4],0,8)MOV(5,Port_Data.Data_Transfer[69])OTL(Local_Control.24);
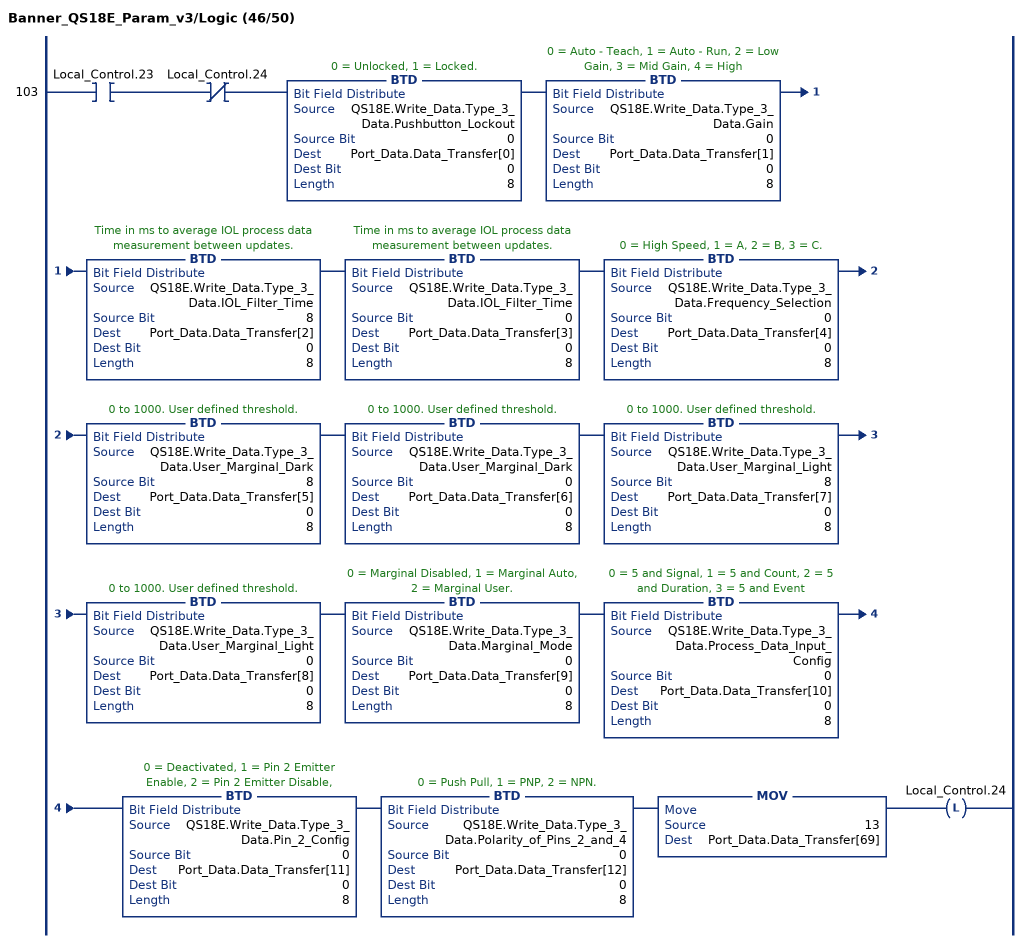
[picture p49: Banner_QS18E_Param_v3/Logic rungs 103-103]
   103: XIC(Local_Control.23)XIO(Local_Control.24)BTD(QS18E.Write_Data.Type_3_Data.Pushbutton_Lockout,0,Port_Data.Data_Transfer[0],0,8)BTD(QS18E.Write_Data.Type_3_Data.Gain,0,Port_Data.Data_Transfer[1],0,8)BTD(QS18E.Write_Data.Type_3_Data.IOL_Filter_Time,8,Port_Data.Data_Transfer[2],0,8)BTD(QS18E.Write_Data.Type_3_Data.IOL_Filter_Time,0,Port_Data.Data_Transfer[3],0,8)BTD(QS18E.Write_Data.Type_3_Data.Frequency_Selection,0,Port_Data.Data_Transfer[4],0,8)BTD(QS18E.Write_Data.Type_3_Data.User_Marginal_Dark,8,Port_Data.Data_Transfer[5],0,8)BTD(QS18E.Write_Data.Type_3_Data.User_Marginal_Dark,0,Port_Data.Data_Transfer[6],0,8)BTD(QS18E.Write_Data.Type_3_Data.User_Marginal_Light,8,Port_Data.Data_Transfer[7],0,8)BTD(QS18E.Write_Data.Type_3_Data.User_Marginal_Light,0,Port_Data.Data_Transfer[8],0,8)BTD(QS18E.Write_Data.Type_3_Data.Marginal_Mode,0,Port_Data.Data_Transfer[9],0,8)BTD(QS18E.Write_Data.Type_3_Data.Process_Data_Input_Config,0,Port_Data.Data_Transfer[10],0,8)BTD(QS18E.Write_Data.Type_3_Data.Pin_2_Config,0,Port_Data.Data_Transfer[11],0,8)BTD(QS18E.Write_Data.Type_3_Data.Polarity_of_Pins_2_and_4,0,Port_Data.Data_Transfer[12],0,8)MOV(13,Port_Data.Data_Transfer[69])OTL(Local_Control.24);
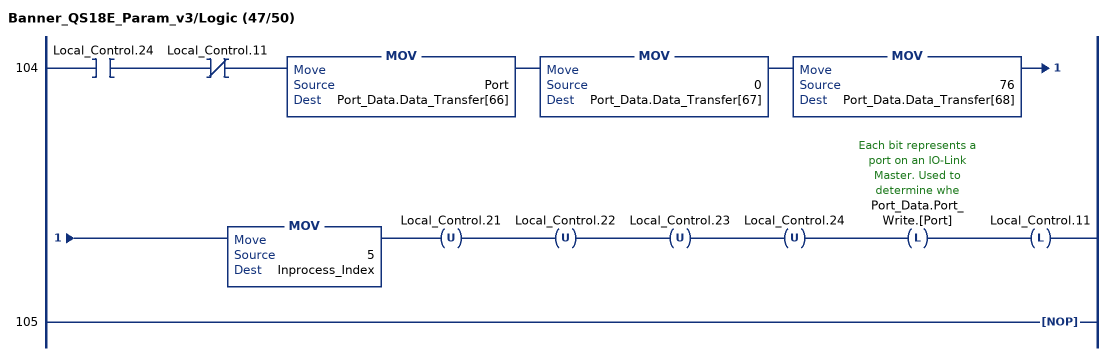
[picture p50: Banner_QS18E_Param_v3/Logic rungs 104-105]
   104: XIC(Local_Control.24)XIO(Local_Control.11)MOV(Port,Port_Data.Data_Transfer[66])MOV(0,Port_Data.Data_Transfer[67])MOV(76,Port_Data.Data_Transfer[68])MOV(5,Inprocess_Index)OTU(Local_Control.21)OTU(Local_Control.22)OTU(Local_Control.23)OTU(Local_Control.24)OTL(Port_Data.Port_Write.[Port])OTL(Local_Control.11);
   105: NOP();
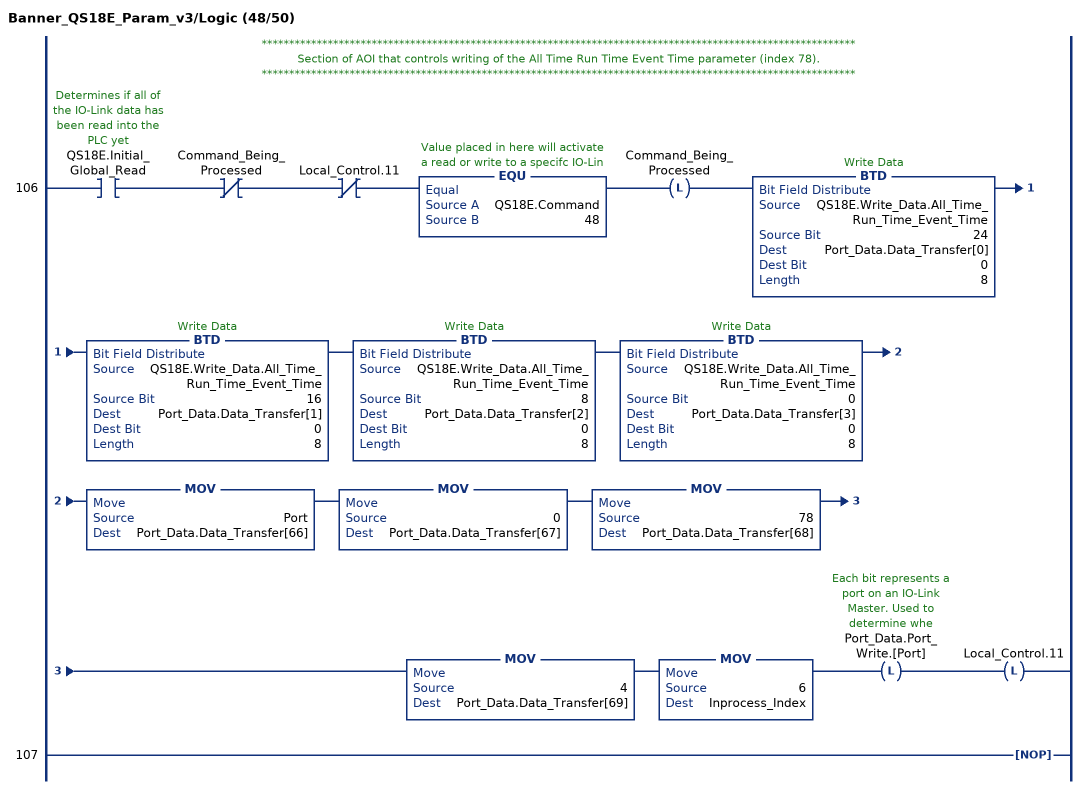
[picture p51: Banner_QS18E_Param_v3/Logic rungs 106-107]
   // ************************************************************************************************************
   // Section of AOI that controls writing of the All Time Run Time Event Time parameter (index 78).
   // ************************************************************************************************************
   106: XIC(QS18E.Initial_Global_Read)XIO(Command_Being_Processed)XIO(Local_Control.11)EQU(QS18E.Command,48)OTL(Command_Being_Processed)BTD(QS18E.Write_Data.All_Time_Run_Time_Event_Time,24,Port_Data.Data_Transfer[0],0,8)BTD(QS18E.Write_Data.All_Time_Run_Time_Event_Time,16,Port_Data.Data_Transfer[1],0,8)BTD(QS18E.Write_Data.All_Time_Run_Time_Event_Time,8,Port_Data.Data_Transfer[2],0,8)BTD(QS18E.Write_Data.All_Time_Run_Time_Event_Time,0,Port_Data.Data_Transfer[3],0,8)MOV(Port,Port_Data.Data_Transfer[66])MOV(0,Port_Data.Data_Transfer[67])MOV(78,Port_Data.Data_Transfer[68])MOV(4,Port_Data.Data_Transfer[69])MOV(6,Inprocess_Index)OTL(Port_Data.Port_Write.[Port])OTL(Local_Control.11);
   107: NOP();
